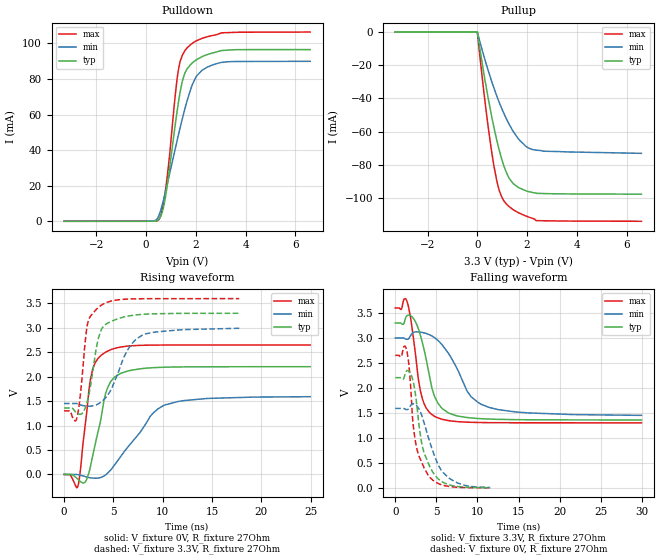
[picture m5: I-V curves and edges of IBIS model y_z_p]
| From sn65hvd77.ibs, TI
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|   y_z Model
[Model]   y_z_p
Model_type   Output
Polarity   Non-Inverting
Vmeas = 1.65
Vref = 1.956
Cref = 50pF
Rref = 27
|   typ   min   max
|   (nom PVT)   (fast PVT)   (slow PVT)
|Avergae
C_comp   1.500e-11   1.433e-11   1.761e-11
| Where nom  PVT is Nominal Process, 3.3V, 27C
|   Fast PVT is Strong Process,  3.6V, -40C
|   Slow PVT is Weak Process,   3V, 150C
[Voltage Range]   3.3   3   3.6
|Ambient Temperature   25   125   -40
|Junction Temperature
[Temperature Range]   27   150   -40
[Pullup Reference]   3.3   3   3.6
[Pulldown Reference]   0   0   0
[Power Clamp Reference]   3.3   3   3.6
[GND Clamp Reference]   0   0   0
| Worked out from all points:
|   slope of the pulldown table from 0 to 0.495 V, typ, clamps not added: 584 ohm
|   slope of the pullup table from 0 to 0.495 V, typ, clamps not added: 11.1 ohm
|   falling waveform, V_fixture 3.3V, R_fixture 27Ohm: 20-80 % time 1.74ns typ, 3.22ns min, 1.26ns max; typ from 3.3 V to 1.36 V
|   rising waveform, V_fixture 0V, R_fixture 27Ohm: 20-80 % time 1.43ns typ, 3.55ns min, 995ps max; typ from 0 V to 2.21 V
|   rising waveform, V_fixture 3.3V, R_fixture 27Ohm: 20-80 % time 1.06ns typ, 2.1ns min, 739ps max; typ from 1.36 V to 3.3 V
|   falling waveform, V_fixture 0V, R_fixture 27Ohm: 20-80 % time 1.61ns typ, 2.18ns min, 1.33ns max; typ from 2.21 V to 0.005 V
[Pulldown]
|   Voltage   I(typ)   I(min)   I(max)
-3.3V     -6.612uA   -9.318uA   -6.374uA
336mV     41.43uA    229.2uA    18.75uA
519.6mV   1.175mA    3.381mA    1.076mA
670.8mV   6.19mA     10.37mA    7.974mA
847.2mV   19.71mA    20.58mA    24.58mA
1.207V    57.83mA    42.86mA    75.34mA
1.311V    67.7mA     49.13mA    85.95mA
1.541V    82.6mA     62.22mA    95.46mA
1.815V    88.49mA    75.13mA    99.61mA
2.253V    92.56mA    84.88mA    102.8mA
3.021V    95.98mA    89.33mA    105.9mA
6.6V      96.55mA    89.94mA    106.4mA
[Pullup]
|   Voltage   I(typ)   I(min)   I(max)
-3.3V     13.22uA    17.2uA     13.33uA
0V        0A         0A         0A
372mV     -34.39mA   -19.93mA   -49.55mA
672mV     -57.7mA    -33.86mA   -80.94mA
816mV     -67.2mA    -39.81mA   -91.73mA
955.2mV   -75.16mA   -45.09mA   -98.48mA
1.155V    -84.1mA    -51.84mA   -103.3mA
1.296V    -88.39mA   -56mA      -105.3mA
1.68V     -93.83mA   -64.82mA   -109mA
2.212V    -96.61mA   -70.72mA   -112.2mA
2.358V    -97mA      -71.09mA   -113.6mA
6.6V      -97.65mA   -73.05mA   -114mA
[Ramp]
R_load = 27
|   typ   min   max
dV/dt_r   1.32345/1.42858e-09   0.954842/3.53984e-09   1.59014/9.90203e-10
dV/dt_f   1.1633/1.7322e-09   0.928432/3.18178e-09   1.37799/1.25238e-09
[Falling Waveform]
V_fixture = 3.3V
V_fixture_min = 3V
V_fixture_max = 3.6V
R_fixture = 27Ohm
|   Time   V(typ)   V(min)   V(max)
0s        3.3V       3V         3.6V
1.39ns    3.439V     2.972V     3.747V
2.44ns    3.328V     3.12V      2.702V
2.84ns    3.171V     3.121V     2.146V
3.315ns   2.893V     3.109V     1.777V
4.855ns   1.808V     2.996V     1.426V
6.445ns   1.503V     2.699V     1.349V
9.22ns    1.401V     1.826V     1.314V
11.39ns   1.379V     1.613V     1.307V
29.95ns   1.361V     1.453V     1.303V
[Rising Waveform]
V_fixture = 0V
V_fixture_min = 0V
V_fixture_max = 0V
R_fixture = 27Ohm
|   Time   V(typ)   V(min)   V(max)
0s        11.31nV    107.3nV    12.29nV
1.39ns    -94.82mV   -4.205mV   -250.5mV
1.655ns   -144.4mV   -16.93mV   78.51mV
2.195ns   -143.5mV   -45.5mV    1.092V
2.585ns   80.85mV    -65.8mV    1.818V
2.885ns   363.1mV    -74.49mV   2.138V
4.385ns   1.757V     18.61mV    2.521V
5.735ns   2.068V     363.6mV    2.608V
10.16ns   2.195V     1.418V     2.649V
24.95ns   2.206V     1.591V     2.65V
[Rising Waveform]
V_fixture = 3.3V
V_fixture_min = 3V
V_fixture_max = 3.6V
R_fixture = 27Ohm
|   Time   V(typ)   V(min)   V(max)
0s        1.36V      1.452V     1.301V
1.26ns    1.267V     1.453V     1.124V
1.565ns   1.233V     1.431V     1.467V
2.075ns   1.325V     1.404V     2.567V
2.585ns   1.698V     1.396V     3.204V
3.285ns   2.601V     1.426V     3.382V
3.815ns   2.979V     1.49V      3.47V
6.425ns   3.239V     2.542V     3.59V
7.905ns   3.276V     2.846V     3.597V
17.77ns   3.299V     2.992V     3.6V
[Falling Waveform]
V_fixture = 0V
V_fixture_min = 0V
V_fixture_max = 0V
R_fixture = 27Ohm
|   Time   V(typ)   V(min)   V(max)
0s        2.206V     1.592V     2.652V
1.31ns    2.328V     1.569V     2.803V
1.65ns    2.334V     1.589V     2.473V
2.135ns   2.162V     1.685V     1.339V
2.42ns    1.915V     1.672V     962.3mV
3.245ns   869.2mV    1.441V     504.6mV
4.025ns   492.1mV    1.011V     252.3mV
5.17ns    192.1mV    480.3mV    95.17mV
6.555ns   63.29mV    196.4mV    30.52mV
11.54ns   5.363mV    10.82mV    3.63mV
